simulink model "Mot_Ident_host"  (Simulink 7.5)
settings: Solver=ode45  StartTime=0.0  StopTime=inf  RelTol=1e-3
undefined symbols (not defined in the file or in its folder): NULL, serial
libraries: instrumentlib x2

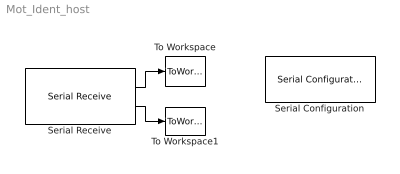
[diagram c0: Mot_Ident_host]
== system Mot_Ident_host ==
  Serial Configuration : instrumentlib/Serial Configuration  Priority=-200000  DialogController=instrumentcreatedialog  DialogControllerArgs=DataTag0  ComPortMenu=<Please select a port...>  ComPort=COM4  ObjConstructor=serial('COM4');  BaudRate=57600  DataBits=8  Parity=none  StopBits=1  FlowControl=none  Timeout=10  ByteOrder=LittleEndian
  Serial Receive : instrumentlib/Serial Receive  DialogController=instrumentcreatedialog  DialogControllerArgs=DataTag1  ComPortMenu=<Please select a port...>  ComPort=COM4  ObjConstructor=serial('COM4');  Header=A  Terminator=NULL ('\0')  DataSize="[1  1]"  DataType=int32  EnableBlockingMode=off  ActionDataUnavailable=Output custom value  CustomValue=0  SampleTime=0.01
  To Workspace : ToWorkspace  VariableName=simout  SampleTime=-1  SaveFormat=Structure With Time
  To Workspace1 : ToWorkspace  VariableName=simout1  SampleTime=-1  SaveFormat=Array
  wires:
  Serial Receive/1 -> To Workspace/1
  Serial Receive/2 -> To Workspace1/1
